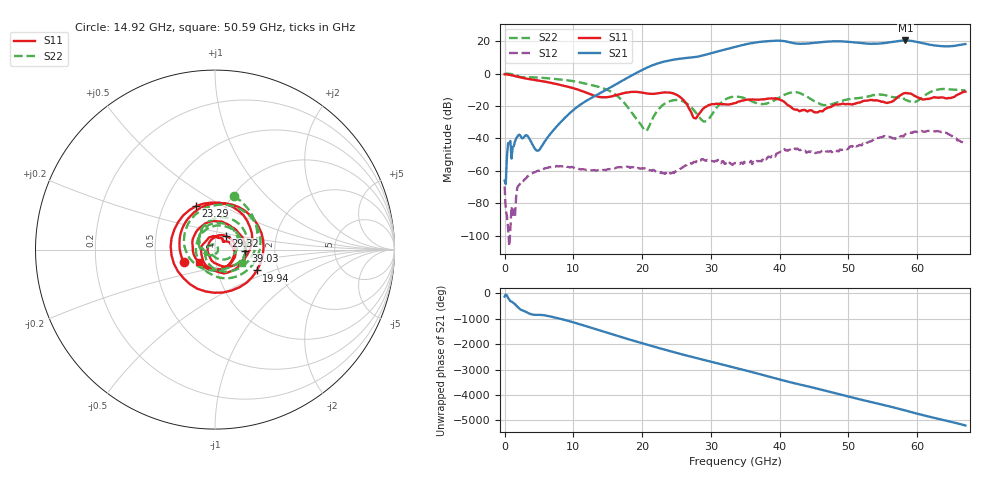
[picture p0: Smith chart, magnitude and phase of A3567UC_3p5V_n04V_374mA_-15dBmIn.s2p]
! MARKI MICROWAVE INC.
! Date:  4/20/2021
! Model Number:  A-3567UC
! Description:  2-port Small Signal S-parameter data for A-3567UC
! Frequency Range:  10 MHz to 67 GHz
! Port Configuration:  PORT 1: Input
!  PORT 2: Output
! Bias Condition: Vd = +3.5V, Vg = -0.4V, Id = 374mA
! A-3567UC s2p files are only valid for small signal conditions (below -10 dBm input power)
# Hz S  dB  R 50
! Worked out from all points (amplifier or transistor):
!   401 points, 10 MHz to 67 GHz, reference 50 ohm
!   highest |S21| = 20.5 dB at 58.29 GHz (marker M1)
!   |S21| within 3 dB of that: 34.45 GHz to 62.38 GHz (27.94 GHz wide, 57.7 % of centre)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
!   unconditionally stable (mu >= 1): 175.7 MHz to end of sweep
!   at 11.06 GHz: K = 2672.88, MAG = -17.2 dB, |S12| = -59.3 dB
!   at 33.51 GHz: K = 40.84, MAG = 16.7 dB, |S12| = -55.2 dB
!   at 67 GHz: K = 7.39, MAG = 19.0 dB, |S12| = -43.1 dB
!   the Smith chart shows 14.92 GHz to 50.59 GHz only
!   S11 on the Smith chart (normalised r, x): 14.92 GHz: 0.70, -0.10; 19.94 GHz: 1.55, -0.39; 23.29 GHz: 0.73, +0.38; 29.32 GHz: 1.11, +0.17; 39.03 GHz: 1.41, -0.02; 50.59 GHz: 0.83, -0.11
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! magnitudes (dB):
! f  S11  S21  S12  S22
! 10 MHz  -0.4  -66.1  -69.7  0.0
! 679.9 MHz  -0.7  -42.9  -106.5  -0.1
! 1.852 GHz  -1.9  -38.9  -70.3  -1.2
! 4.867 GHz  -4.2  -47.5  -59.9  -2.4
! 11.23 GHz  -10.7  -18.5  -59.0  -5.6
! 14.92 GHz  -14.5  -9.7  -59.1  -10.0
! 19.94 GHz  -11.7  2.1  -58.4  -32.4
! 20.78 GHz  -12.3  3.9  -59.3  -34.5
! 22.45 GHz  -12.0  6.6  -60.6  -21.7
! 23.29 GHz  -11.6  7.5  -61.8  -18.5
! 25.63 GHz  -14.8  9.3  -58.6  -16.7
! 27.64 GHz  -27.4  10.2  -54.7  -23.2
! 29.32 GHz  -20.4  11.8  -53.8  -29.2
! 33.51 GHz  -18.2  16.5  -55.2  -14.2
! 39.03 GHz  -15.4  20.3  -51.1  -16.9
! 42.05 GHz  -21.9  18.8  -46.8  -11.4
! 44.73 GHz  -22.9  18.9  -48.8  -16.2
! 50.59 GHz  -19.1  19.4  -44.7  -15.4
! 55.95 GHz  -17.8  19.3  -39.0  -14.1
! 58.29 GHz  -12.0  20.5  -37.3  -16.1
! 63.32 GHz  -14.7  17.1  -35.7  -9.6
! 67 GHz  -11.1  18.3  -43.1  -10.3
